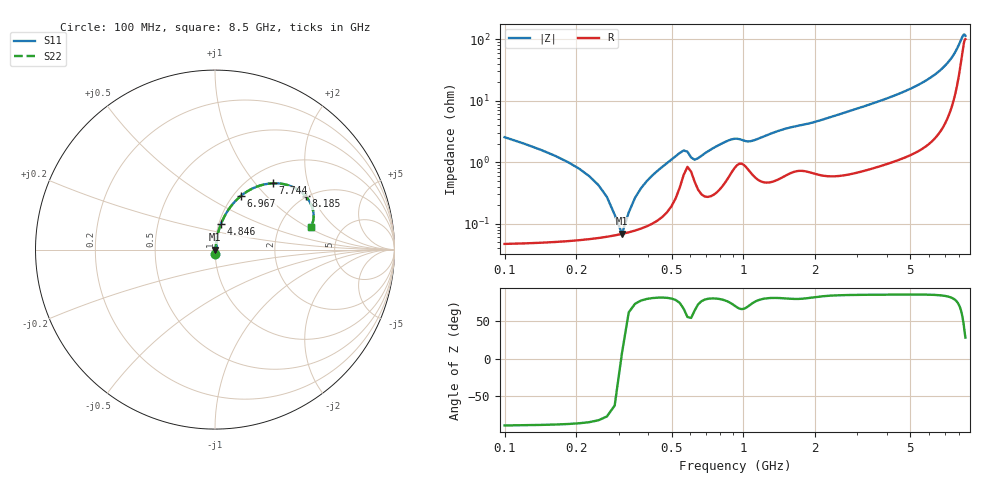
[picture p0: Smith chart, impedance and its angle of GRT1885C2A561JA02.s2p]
!Murata Part Number: GRT1885C2A561JA02
!These Parameters are Measured in Series Mode Connection
!Data Generated on Jun 19, 2026
!  o--ll--o
!Port1  Port2
!  o------o
!Operation Temp=25[degC], DC Bias Voltage=0[V]
!Freq. Start=100[MHz] Stop=9[GHz] 401[Steps]
# Hz S RI R 50
!Freq.(Hz) S11(Real) S11(Imag) S21(Real) S21(Imag) S12(Real) S12(Imag) S22(Real) S22(Imag)
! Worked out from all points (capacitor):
!   401 points, 100 MHz to 8.5 GHz, reference 50 ohm
!   read as one part in series: C = 556 pF near 142 MHz
!   lowest |Z| = 69 mohm at 310 MHz (marker M1)
!   series resonance near 308.6 MHz, so ESL is about 480 pH
!   S11 on the Smith chart (normalised r, x): 100 MHz: 1.00, -0.05; 4.846 GHz: 1.02, +0.29; 6.967 GHz: 1.08, +0.73; 7.744 GHz: 1.28, +1.25; 8.185 GHz: 1.96, +1.78; 8.5 GHz: 3.00, +1.06
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1e8  0.00112 -0.0255  0.9989 0.0255  0.9989 0.0255  0.00112 -0.0255
1.84e8  0.000623 -0.01  0.9994 0.01  0.9994 0.01  0.000623 -0.01
2.26e8  0.000597 -0.00592  0.9994 0.00592  0.9994 0.00592  0.000597 -0.00592
2.68e8  0.000622 -0.00267  0.9994 0.00267  0.9994 0.00267  0.000622 -0.00267
3.1e8  0.000684 8.68e-05  0.9993 -8.68e-05  0.9993 -8.68e-05  0.000684 8.68e-05
3.52e8  0.000783 0.00255  0.9992 -0.00255  0.9992 -0.00255  0.000783 0.00255
3.73e8  0.00085 0.00371  0.9991 -0.00371  0.9991 -0.00371  0.00085 0.00371
4.15e8  0.00104 0.00598  0.999 -0.00598  0.999 -0.00598  0.00104 0.00598
5.41e8  0.00402 0.0135  0.996 -0.0135  0.996 -0.0135  0.00402 0.0135
6.46e8  0.00369 0.011  0.9963 -0.011  0.9963 -0.011  0.00369 0.011
8.77e8  0.00658 0.0219  0.9934 -0.0219  0.9934 -0.0219  0.00658 0.0219
1.087e9  0.00677 0.021  0.9932 -0.021  0.9932 -0.021  0.00677 0.021
1.507e9  0.00725 0.0343  0.9928 -0.0343  0.9928 -0.0343  0.00725 0.0343
2.914e9  0.0116 0.0703  0.9884 -0.0703  0.9884 -0.0703  0.0116 0.0703
4.3e9  0.0243 0.1171  0.9757 -0.1171  0.9757 -0.1171  0.0243 0.1171
4.846e9  0.0326 0.1407  0.9674 -0.1407  0.9674 -0.1407  0.0326 0.1407
5.707e9  0.0547 0.1888  0.9453 -0.1888  0.9453 -0.1888  0.0547 0.1888
6.967e9  0.1446 0.2992  0.8554 -0.2992  0.8554 -0.2992  0.1446 0.2992
7.114e9  0.1663 0.3155  0.8337 -0.3155  0.8337 -0.3155  0.1663 0.3155
7.744e9  0.324 0.3694  0.676 -0.3694  0.676 -0.3694  0.324 0.3694
8.185e9  0.5045 0.2982  0.4955 -0.2982  0.4955 -0.2982  0.5045 0.2982
8.5e9  0.5333 0.124  0.4667 -0.124  0.4667 -0.124  0.5333 0.124
